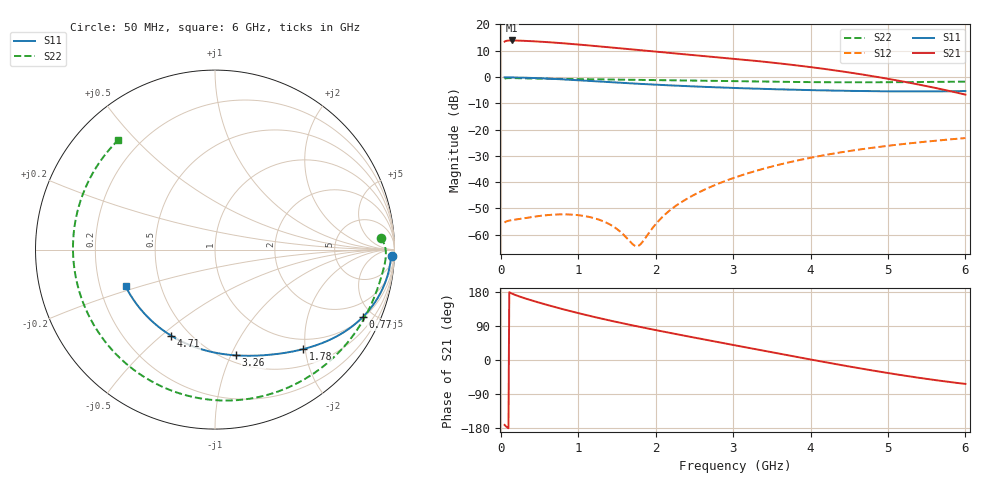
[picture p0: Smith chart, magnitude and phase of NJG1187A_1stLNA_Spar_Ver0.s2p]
! Created Wed Mar 10 19:48:52 2021
# hz S ma R 50
! 2 Port Network Data from SP11.SP block
! freq  magS11  angS11  magS21  angS21  magS12  angS12  magS22  angS22
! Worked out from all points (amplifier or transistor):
!   596 points, 50 MHz to 6 GHz, reference 50 ohm
!   highest |S21| = 13.9 dB at 140 MHz (marker M1)
!   |S21| within 3 dB of that: start of sweep to 1.547 GHz
!   unconditionally stable (mu >= 1): start of sweep to end of sweep
!   at 1.04 GHz: K = 3.05, MAG = 24.7 dB, |S12| = -52.7 dB
!   at 3.03 GHz: K = 3.04, MAG = 14.8 dB, |S12| = -38.2 dB
!   at 6 GHz: K = 3.69, MAG = -0.3 dB, |S12| = -23.2 dB
!   lowest NFmin = 0.25 dB at 50 MHz
!   S11 on the Smith chart (normalised r, x): 50 MHz: 20, -46; 770 MHz: 1.05, -4.34; 1.78 GHz: 0.80, -1.96; 3.26 GHz: 0.57, -1.04; 4.71 GHz: 0.40, -0.54; 6 GHz: 0.31, -0.18
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5e7  0.9845 -2.1  4.698 -171.4  0.0017 29.9  0.9252 4.0
9e7  0.9815 -3.3  4.901 -178.7  0.00183 21.4  0.9492 0.5
1.4e8  0.979 -4.9  4.939 175.7  0.001893 19.1  0.9524 -2.3
2.6e8  0.9713 -8.9  4.89 166.3  0.002017 20.9  0.9444 -6.9
4.2e8  0.9555 -14.1  4.767 156.0  0.002195 25.1  0.9343 -11.6
5.9e8  0.933 -19.4  4.605 145.9  0.002355 28.2  0.9266 -16.3
7.7e8  0.9046 -24.6  4.408 135.8  0.00244 29.9  0.9197 -21.3
1.05e9  0.8566 -32.1  4.076 121.3  0.002307 31.1  0.9096 -29.1
1.38e9  0.801 -39.9  3.685 105.5  0.001654 35.0  0.8977 -38.6
1.71e9  0.7511 -46.9  3.323 91.0  0.0006494 79.1  0.8856 -48.6
1.78e9  0.7414 -48.4  3.251 88.1  0.0006196 111.2  0.8829 -50.8
2.04e9  0.7082 -53.6  3 77.4  0.001845 167.1  0.8729 -59.4
2.52e9  0.6576 -63.1  2.589 58.3  0.005987 173.7  0.8532 -76.6
3.03e9  0.6162 -73.7  2.206 38.6  0.01235 167.6  0.8313 -97.4
3.26e9  0.6007 -78.8  2.043 29.7  0.01583 164.0  0.8217 -107.5
3.62e9  0.5799 -87.3  1.795 15.8  0.02194 157.6  0.8081 -124.3
4.02e9  0.5609 -97.4  1.526 0.6  0.02948 150.1  0.7968 -143.7
4.36e9  0.5481 -106.7  1.305 -12.0  0.03623 143.6  0.7916 -160.4
4.71e9  0.5383 -116.9  1.089 -24.6  0.0433 137.1  0.7909 -177.1
5.01e9  0.533 -126.0  0.917 -34.7  0.04933 131.8  0.7936 169.3
5.52e9  0.5313 -142.2  0.6596 -50.5  0.05945 123.6  0.8031 148.4
6e9  0.5388 -157.7  0.4616 -63.1  0.06896 116.8  0.8145 131.4
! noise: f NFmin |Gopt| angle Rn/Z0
5e+07  0.2541  0.9655  5.166  1.694
7.1e+08  0.3207  0.8072  18.5  0.324
1.37e+09  0.4817  0.7356  34.02  0.3063
2.03e+09  0.7187  0.6538  51.12  0.2888
2.69e+09  1.044  0.5706  70.08  0.2667
3.35e+09  1.488  0.4939  91.2  0.2423
4.01e+09  2.109  0.4325  114.2  0.2229
4.67e+09  2.992  0.3942  137.7  0.2226
5.33e+09  4.269  0.3827  159.3  0.2657
6e+09  6.188  0.3992  177.2  0.405
